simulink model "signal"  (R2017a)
settings: Solver=FixedStepDiscrete  StartTime=0.0  StopTime=inf  RelTol=1e-3  EnableMultiTasking=on
undefined symbols (not defined in the file): ADCIN0, ADCIN1, ADCINA0, ADCINB0, bit, ended, input, Single
libraries: c2802xlib x1, c280xlib x1

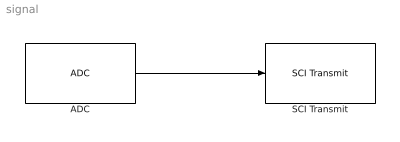
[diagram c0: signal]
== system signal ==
  ADC : c2802xlib/ADC  ADCModule=A  samplingMode=Single sample mode  ADCResolution=12-bit (Single-ended input)  useSOC1=SOC0  useSOC2=SOC0_SOC1  SOCAcquisitionWindow=7  SOCTriggerSource=Software  SOCInterruptTrigger=No ADCINT  Ts=0.1  dType=uint16  postInterrupt=off  interruptSel=ADCINT1  ADCINTContinuous=on  endma=off  chdma=1  blkParamProc=C2000_Type4  conv1=ADCINA0  conv2=ADCINA0 and ADCINB0  conv1_Type4=ADCIN2  conv2_Type4=ADCIN0 and ADCIN1
  SCI Transmit : c280xlib/SCI Transmit  sciModule=A  dataHead='S'  dataTail='E'  postInterrupt=off  numFifo=1
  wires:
  ADC/1 -> SCI Transmit/1
